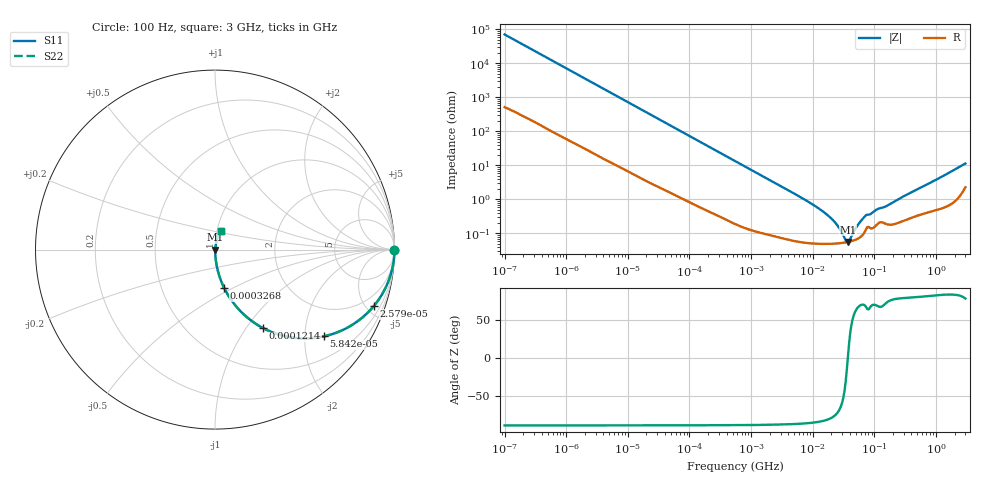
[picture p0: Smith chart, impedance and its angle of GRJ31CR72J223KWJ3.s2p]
!Murata Part Number: GRJ31CR72J223KWJ3
!These Parameters are Measured in Series Mode Connection
!Data Generated on Jun 19, 2026
!  o--ll--o
!Port1  Port2
!  o------o
!Operation Temp=25[degC], DC Bias Voltage=0[V]
!Freq. Start=100[Hz] Stop=3[GHz] 401[Steps]
# Hz S RI R 50
!Freq.(Hz) S11(Real) S11(Imag) S21(Real) S21(Imag) S12(Real) S12(Imag) S22(Real) S22(Imag)
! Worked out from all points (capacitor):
!   401 points, 100 Hz to 3 GHz, reference 50 ohm
!   read as one part in series: C = 22.6 nF near 109 Hz
!   lowest |Z| = 55.6 mohm at 37.19 MHz (marker M1)
!   series resonance near 37.12 MHz, so ESL is about 810 pH
!   S11 on the Smith chart (normalised r, x): 100 Hz: open; 25.79 kHz: 1.05, -5.62; 58.42 kHz: 1.03, -2.50; 121.4 kHz: 1.01, -1.21; 326.8 kHz: 1.01, -0.45; 3 GHz: 1.05, +0.22
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100  1 -0.00142  1.24e-05 0.00142  1.24e-05 0.00142  1 -0.00142
1788  0.9992 -0.025  0.000841 0.025  0.000841 0.025  0.9992 -0.025
8066  0.9866 -0.1103  0.0134 0.1103  0.0134 0.1103  0.9866 -0.1103
25785  0.8854 -0.3137  0.1146 0.3137  0.1146 0.3137  0.8854 -0.3137
31977  0.8351 -0.3661  0.1649 0.3661  0.1649 0.3661  0.8351 -0.3661
58416  0.6079 -0.4829  0.3921 0.4829  0.3921 0.4829  0.6079 -0.4829
121426  0.2692 -0.4379  0.7308 0.4379  0.7308 0.4379  0.2692 -0.4379
194955  0.1275 -0.3274  0.8725 0.3274  0.8725 0.3274  0.1275 -0.3274
326774  0.0511 -0.2137  0.9489 0.2137  0.9489 0.2137  0.0511 -0.2137
547723  0.0197 -0.1323  0.9803 0.1323  0.9803 0.1323  0.0197 -0.1323
1677156  0.00292 -0.0442  0.9971 0.0442  0.9971 0.0442  0.00292 -0.0442
9794414  0.000555 -0.00718  0.9994 0.00718  0.9994 0.00718  0.000555 -0.00718
1.572531e7  0.000503 -0.00395  0.9995 0.00395  0.9995 0.00395  0.000503 -0.00395
2.12544e7  0.0005 -0.0024  0.9995 0.0024  0.9995 0.0024  0.0005 -0.0024
2.635803e7  0.00051 -0.00143  0.9995 0.00143  0.9995 0.00143  0.00051 -0.00143
3.412477e7  0.00054 -0.000346  0.9995 0.000346  0.9995 0.000346  0.00054 -0.000346
3.71925e7  0.000556 8.5e-06  0.9994 -8.5e-06  0.9994 -8.5e-06  0.000556 8.5e-06
4.0536e7  0.000576 0.000365  0.9994 -0.000365  0.9994 -0.000365  0.000576 0.000365
5.478864e7  0.000709 0.00168  0.9993 -0.00168  0.9993 -0.00168  0.000709 0.00168
7.093284e7  0.00117 0.003  0.9988 -0.003  0.9988 -0.003  0.00117 0.003
1.751444e8  0.00183 0.00684  0.9982 -0.00684  0.9982 -0.00684  0.00183 0.00684
3e9  0.0334 0.1046  0.9666 -0.1046  0.9666 -0.1046  0.0334 0.1046
